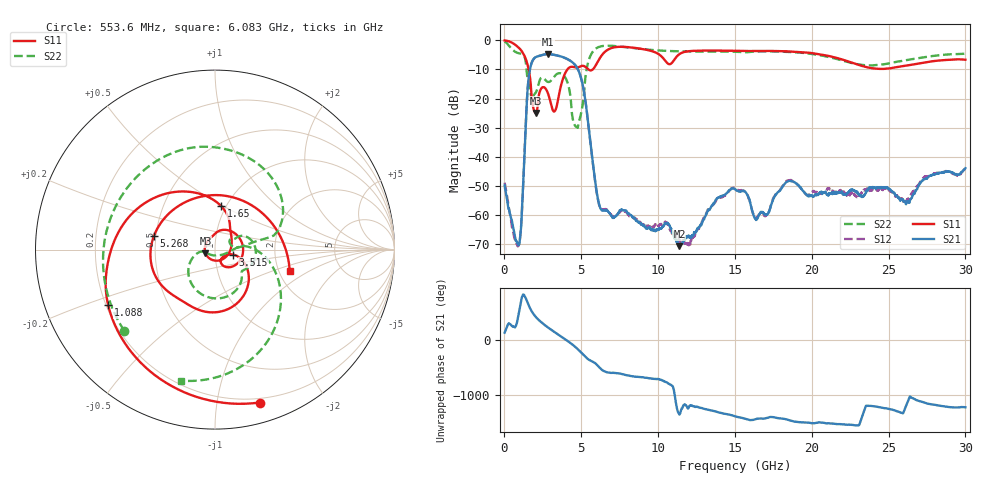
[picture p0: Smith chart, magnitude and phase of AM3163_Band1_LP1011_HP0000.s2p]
!Agilent Technologies,E8364B,MY43040894,A.07.50.67
!Agilent E8364B: A.07.50.67
!Date: Thursday, August 20, 2020 11:29:22
!Correction: S11(Full 2 Port(1,2))
!S21(Full 2 Port(1,2))
!S12(Full 2 Port(1,2))
!S22(Full 2 Port(1,2))
!S2P File: Measurements: S11, S21, S12, S22:
# Hz S  dB  R 50
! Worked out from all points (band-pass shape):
!   3201 points, 10 MHz to 30 GHz, reference 50 ohm
!   highest |S21| = -4.79 dB at 2.812 GHz (marker M1); lowest = -70.6 dB at 11.39 GHz (marker M2)
!   |S21| within 3 dB of the highest: 1.768 GHz to 4.47 GHz (2.702 GHz wide, 86.6 % of centre)
!   lowest |S11| = -24.9 dB at 2.025 GHz (marker M3), VSWR 1.12, Z = 44.9 - j1.79 ohm
!   |S11| at or under -10 dB: 1.575 GHz to 4.1 GHz (2.525 GHz wide, 89 % of centre); 5.456 GHz to 5.752 GHz (296.2 MHz wide, 5.29 % of centre)
!   |S22| runs from -30.1 to -0.4 dB; largest |S21 - S12| = 0.0057
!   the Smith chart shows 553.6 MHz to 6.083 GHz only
!   S11 on the Smith chart (normalised r, x): 553.6 MHz: 0.16, -1.32; 1.088 GHz: 0.21, -0.23; 1.65 GHz: 0.95, +0.49; 3.515 GHz: 1.22, -0.07; 5.268 GHz: 0.49, +0.08; 6.083 GHz: 2.29, -0.67
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1e7  -0.08 -9.1  -49.85 124.7  -48.86 -123.0  -0.42 -19.3
5.535688e8  -1.04 -73.8  -63.80 -128.6  -65.29 -125.5  -3.37 -138.2
1.087766e9  -3.47 -152.6  -63.67 -24.4  -63.46 131.1  -4.63 111.2
1.650078e9  -12.27 81.6  -10.29 -147.9  -10.29 -148.0  -16.77 6.1
2.024953e9  -24.95 -159.5  -5.84 52.4  -5.84 52.4  -18.07 28.7
2.812191e9  -17.95 -50.9  -4.79 -138.0  -4.79 -138.0  -14.28 -36.9
3.515081e9  -19.66 -15.5  -5.33 87.7  -5.35 87.7  -11.34 -78.7
4.349178e9  -9.12 -91.6  -7.29 -73.5  -7.27 -73.3  -22.74 -171.9
5.014581e9  -8.84 -151.8  -13.57 120.4  -13.54 120.4  -24.38 -22.4
5.267622e9  -9.15 167.8  -20.73 48.5  -20.72 48.2  -12.67 -1.1
6.082975e9  -7.27 -16.0  -54.37 -112.9  -54.70 -112.3  -2.45 -104.5
6.776494e9  -3.10 -103.2  -58.92 125.7  -58.92 124.1  -1.88 -155.4
7.760541e9  -2.27 -173.8  -58.35 92.7  -58.46 93.4  -2.31 153.4
1.000979e10  -4.69 75.0  -64.84 9.0  -63.65 1.6  -3.50 62.5
1.138746e10  -4.77 54.0  -70.63 90.6  -68.84 -95.2  -3.80 13.5
1.5005e10  -3.63 -71.8  -51.11 59.3  -50.63 61.2  -3.95 -93.2
1.636392e10  -3.67 -104.5  -61.51 8.2  -61.10 10.8  -3.88 -124.3
2.000958e10  -4.42 163.5  -53.27 -64.1  -52.25 -56.6  -4.70 136.5
2.275554e10  -7.99 60.4  -51.53 -99.7  -52.91 -99.8  -8.00 21.2
2.500479e10  -9.69 -62.2  -50.93 -167.8  -51.29 -171.4  -7.98 -92.3
2.756331e10  -7.44 -170.2  -47.01 -73.1  -46.65 -70.8  -5.64 175.2
3e10  -6.70 104.7  -43.90 -137.2  -44.14 -131.5  -4.63 102.4
